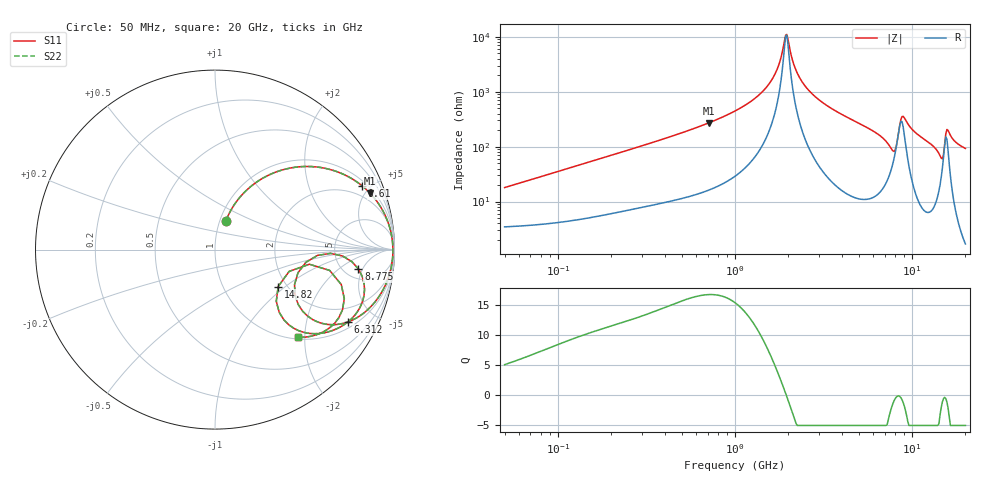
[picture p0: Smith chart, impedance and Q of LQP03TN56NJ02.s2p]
!Murata Part Number: LQP03TN56NJ02
!These Parameters are Measured in Series Mode Connection
!  o--[Z]--o
!Port1  Port2
!  o-------o
!Freq. Start=50[MHz] Stop=20[GHz], 401[Steps]
# Hz S RI R 50
!Freq.(Hz) S11(Real) S11(Imag) S21(Real) S21(Imag) S12(Real) S12(Imag) S22(Real) S22(Imag)
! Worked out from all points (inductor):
!   401 points, 50 MHz to 20 GHz, reference 50 ohm
!   read as one part in series: L = 56 nH near 51.52 MHz
!   highest Q = 16.8 at 708.6 MHz (marker M1), where L = 60.6 nH
!   self-resonance near 1.933 GHz
!   S11 on the Smith chart (normalised r, x): 50 MHz: 1.07, +0.35; 610 MHz: 1.27, +4.48; 6.312 GHz: 1.26, -3.49; 8.775 GHz: 6.72, -4.15; 14.82 GHz: 1.80, -0.89; 20 GHz: 1.03, -1.86
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5e7  0.0608 0.1604  0.9392 -0.1604  0.9392 -0.1604  0.0608 0.1604
1.364002e8  0.2092 0.3595  0.7908 -0.3595  0.7908 -0.3595  0.2092 0.3595
3.721004e8  0.6204 0.4514  0.3796 -0.4514  0.3796 -0.4514  0.6204 0.4514
6.100003e8  0.82 0.355  0.18 -0.355  0.18 -0.355  0.82 0.355
7.08568e8  0.8653 0.3128  0.1347 -0.3128  0.1347 -0.3128  0.8653 0.3128
1e9  0.94 0.2072  0.06 -0.2072  0.06 -0.2072  0.94 0.2072
1.567309e9  0.9856 0.0674  0.0144 -0.0674  0.0144 -0.0674  0.9856 0.0674
1.740566e9  0.9896 0.0351  0.0104 -0.0351  0.0104 -0.0351  0.9896 0.0351
1.932977e9  0.9912 0.00271  0.00881 -0.00271  0.00881 -0.00271  0.9912 0.00271
2.279204e9  0.9892 -0.0486  0.0108 0.0486  0.0108 0.0486  0.9892 -0.0486
2.728004e9  0.9801 -0.1059  0.0199 0.1059  0.0199 0.1059  0.9801 -0.1059
6.311513e9  0.7388 -0.4036  0.2612 0.4036  0.2612 0.4036  0.7388 -0.4036
7.442007e9  0.5165 -0.371  0.4835 0.371  0.4835 0.371  0.5165 -0.371
8.020766e9  0.4622 -0.1293  0.5378 0.1293  0.5378 0.1293  0.4622 -0.1293
8.774992e9  0.7991 -0.108  0.2009 0.108  0.2009 0.108  0.7991 -0.108
1.004137e10  0.7817 -0.3619  0.2183 0.3619  0.2183 0.3619  0.7817 -0.3619
1.220001e10  0.6019 -0.4646  0.3981 0.4646  0.3981 0.4646  0.6019 -0.4646
1.375312e10  0.4402 -0.4391  0.5598 0.4391  0.5598 0.4391  0.4402 -0.4391
1.482269e10  0.3519 -0.2058  0.6481 0.2058  0.6481 0.2058  0.3519 -0.2058
1.550395e10  0.6389 -0.1161  0.3611 0.1161  0.3611 0.1161  0.6389 -0.1161
1.621653e10  0.7107 -0.3346  0.2893 0.3346  0.2893 0.3346  0.7107 -0.3346
2e10  0.4639 -0.4897  0.5361 0.4897  0.5361 0.4897  0.4639 -0.4897
